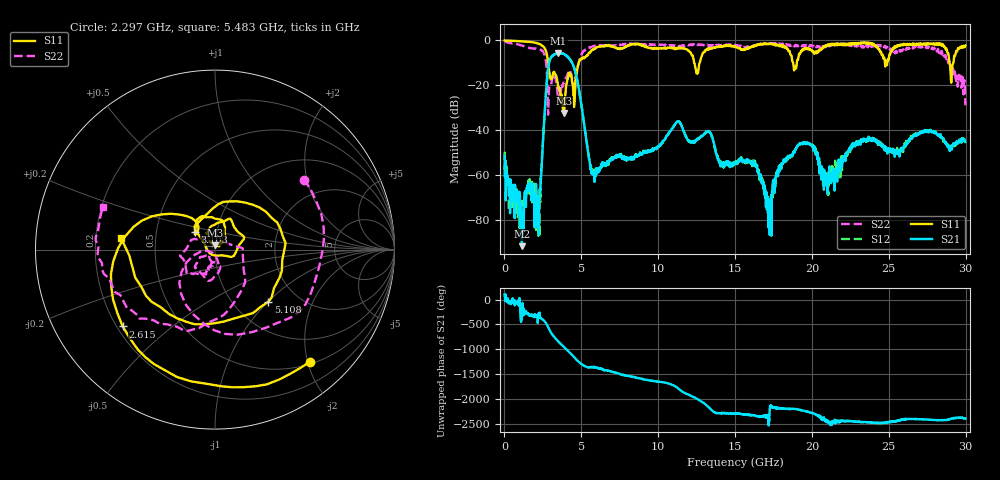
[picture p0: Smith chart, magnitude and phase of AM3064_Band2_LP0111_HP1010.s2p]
# Hz S DB R 50.0
!freq dBS11 angS11 dBS21 angS21 dBS12 angS12 dBS22 angS22
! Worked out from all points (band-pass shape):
!   1600 points, 10 MHz to 29.98 GHz, reference 50 ohm
!   highest |S21| = -5.56 dB at 3.515 GHz (marker M1); lowest = -91.4 dB at 1.135 GHz (marker M2)
!   |S21| within 3 dB of the highest: 2.964 GHz to 4.265 GHz (1.301 GHz wide, 36 % of centre)
!   lowest |S11| = -32.2 dB at 3.871 GHz (marker M3), VSWR 1.05, Z = 50.1 + j2.45 ohm
!   |S11| at or under -10 dB: 2.84 GHz to 4.834 GHz (1.993 GHz wide, 51.9 % of centre); 12.35 GHz to 12.7 GHz (351 MHz wide, 2.8 % of centre); 28.94 GHz to 29.2 GHz (256 MHz wide, 0.881 % of centre)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
!   |S22| runs from -33.0 to -0.2 dB; largest |S21 - S12| = 0.016
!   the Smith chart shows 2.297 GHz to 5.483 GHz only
!   S11 on the Smith chart (normalised r, x): 2.297 GHz: 0.54, -2.05; 2.615 GHz: 0.22, -0.35; 3.103 GHz: 0.78, +0.16; 5.108 GHz: 1.43, -1.00; 5.483 GHz: 0.31, +0.06
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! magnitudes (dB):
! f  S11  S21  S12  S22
! 10 MHz  0.0  -51.3  -49.4  -0.2
! 1.135 GHz  -0.5  -91.4  -75.3  -2.2
! 2.297 GHz  -1.7  -68.2  -66.2  -4.0
! 2.615 GHz  -3.5  -32.1  -32.2  -6.5
! 3.103 GHz  -16.5  -6.9  -7.0  -17.3
! 3.515 GHz  -20.8  -5.6  -5.8  -27.2
! 3.871 GHz  -32.2  -6.1  -6.0  -18.8
! 5.015 GHz  -8.4  -29.4  -29.3  -6.4
! 5.108 GHz  -7.6  -33.5  -33.6  -4.9
! 5.483 GHz  -5.6  -51.4  -51.5  -3.5
! 10 GHz  -3.6  -46.9  -46.9  -2.0
! 11.31 GHz  -3.2  -36.0  -36.0  -2.6
! 15 GHz  -2.6  -54.5  -55.1  -2.0
! 16.32 GHz  -2.3  -56.1  -54.6  -2.2
! 17.22 GHz  -1.4  -74.1  -77.7  -1.5
! 18.17 GHz  -2.7  -52.8  -53.2  -2.1
! 19.99 GHz  -4.3  -46.6  -46.6  -2.2
! 20.93 GHz  -2.3  -59.8  -60.8  -2.3
! 25 GHz  -8.3  -49.2  -49.7  -3.2
! 28.31 GHz  -1.9  -42.8  -42.2  -4.7
! 29.06 GHz  -18.8  -47.6  -47.2  -11.9
! 29.98 GHz  -2.3  -45.2  -44.8  -28.9
